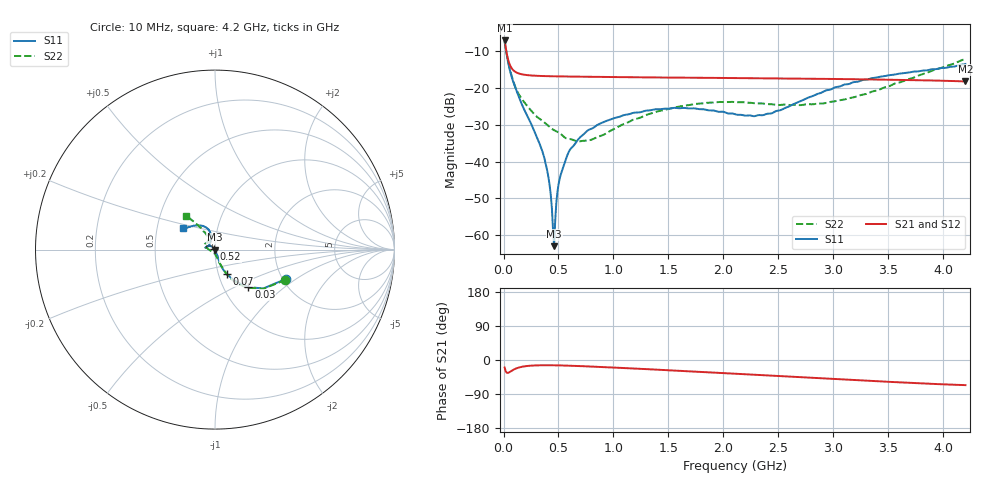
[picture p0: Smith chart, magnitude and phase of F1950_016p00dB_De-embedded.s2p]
! Integrated Device Technology
! Corporate Headquarters
! 6024 Silver Creek Valley Road
! San Jose, CA 95138  USA
! Phone:  1-408-284-8200
! Toll Free:  1-800-223-1366
! Webpage:  http://www.idt.com/
! Timing and RF Division
! 515 Groton Road, Suite 102
! Westford, MA 01886-6024
! Device:  F1950
! Description: 7-bit 0.25 dB Digital Step Attenuator
! Frequency:  150.0 -  4000.00 MHz
! Package:  4x4 mm Thin QFN Plastic Package: 24 pin
! Ports:  2 RF, 12 DC
!  Pin  1  = D0
!  Pin  2  = VDD
!  Pin  3  = Vmode
!  Pin  4  = GND
!  Pin  5  = RF1  =  Port 1
!  Pin  6  = GND
!  Pin  7  = GND
!  Pin  8  = GND
!  Pin  9  = GND
!  Pin 10  = GND
!  Pin 11  = GND
!  Pin 12  = GND
!  Pin 13  = GND
!  Pin 14  = RF2  =  Port 2
!  Pin 15  = GND
!  Pin 16  = LE
!  Pin 17  = CLK
!  Pin 18  = DATE
!  Pin 19  = D6
!  Pin 20  = D5
!  Pin 21  = D4
!  Pin 22  = D3
!  Pin 23  = D2
!  Pin 24  = D1
! State:  64
! Atten State:  16.00 dB
! Voltage:  +5.00 Volts
! Current:  Not Measured mA
! Data:  The device was measured on a the F195X evaluation board which has
!  individual transmission lines to the RF pins.  Data was collected
!  using a calibrated network analyzer.  The evaluation board was
!  de-embedded using a TRL calibration technique.
!  The reference plane is the edge of the package pin.
! Misc:  Board 2019
!  Action Tracker AT0250
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# GHz S dB R 50
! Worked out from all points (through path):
!   420 points, 10 MHz to 4.2 GHz, reference 50 ohm
!   highest |S21| = -7.07 dB at 10 MHz (marker M1); lowest = -18.2 dB at 4.2 GHz (marker M2)
!   group delay of S21, straight-line fit = 37.2 ps
!   lowest |S11| = -62.9 dB at 460 MHz (marker M3), VSWR 1.00, Z = 49.9 - j0.0118 ohm
!   |S11| at or under -10 dB: 24.14 MHz to end of sweep
!   |S22| runs from -34.5 to -7.4 dB; largest |S21 - S12| = 0.0002
!   S11 on the Smith chart (normalised r, x): 10 MHz: 2.07, -0.83; 30 MHz: 1.31, -0.59; 70 MHz: 1.09, -0.30; 520 MHz: 0.99, +0.01; 4.2 GHz: 0.68, +0.17
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0.01  -7.41 -22.7  -7.07 -19.9  -7.07 -19.9  -7.39 -23.3
0.03  -11.08 -48.3  -10.71 -33.8  -10.71 -33.8  -10.98 -48.9
0.07  -16.54 -64.4  -14.43 -29.1  -14.43 -29.1  -16.26 -64.4
0.16  -23.95 -70.6  -16.22 -18.4  -16.21 -18.4  -22.69 -72.3
0.36  -37.85 -65.2  -16.74 -13.8  -16.74 -13.8  -29.05 -80.9
0.41  -44.49 -69.1  -16.78 -13.8  -16.78 -13.8  -30.32 -82.6
0.42  -46.51 -71.7  -16.79 -13.8  -16.79 -13.9  -30.58 -83.5
0.44  -52.67 -80.4  -16.80 -13.9  -16.80 -13.9  -31.07 -86.0
0.46  -62.95 -170.5  -16.81 -14.0  -16.81 -14.0  -31.45 -89.0
0.47  -56.08 143.9  -16.82 -14.0  -16.82 -14.0  -31.60 -90.4
0.5  -46.25 132.4  -16.83 -14.2  -16.83 -14.2  -32.04 -93.2
0.52  -43.55 133.2  -16.84 -14.4  -16.84 -14.4  -32.44 -94.4
0.6  -36.95 133.3  -16.88 -15.0  -16.88 -15.1  -33.84 -108.5
0.71  -33.04 136.5  -16.91 -16.2  -16.91 -16.2  -34.39 -127.5
0.99  -28.36 147.1  -17.01 -19.8  -17.01 -19.8  -31.36 -169.5
1.41  -25.75 163.6  -17.12 -25.7  -17.12 -25.7  -26.27 168.4
1.73  -25.50 169.3  -17.20 -30.4  -17.20 -30.4  -24.37 159.9
2.11  -27.15 159.3  -17.29 -36.3  -17.29 -36.3  -23.84 150.8
2.43  -26.93 127.3  -17.37 -41.1  -17.37 -41.1  -24.38 141.6
2.81  -22.18 105.8  -17.48 -47.1  -17.47 -47.1  -24.42 127.1
3.51  -16.50 117.8  -17.73 -57.7  -17.72 -57.7  -19.47 120.5
4.2  -13.47 146.4  -18.21 -66.3  -18.20 -66.4  -12.09 130.3
